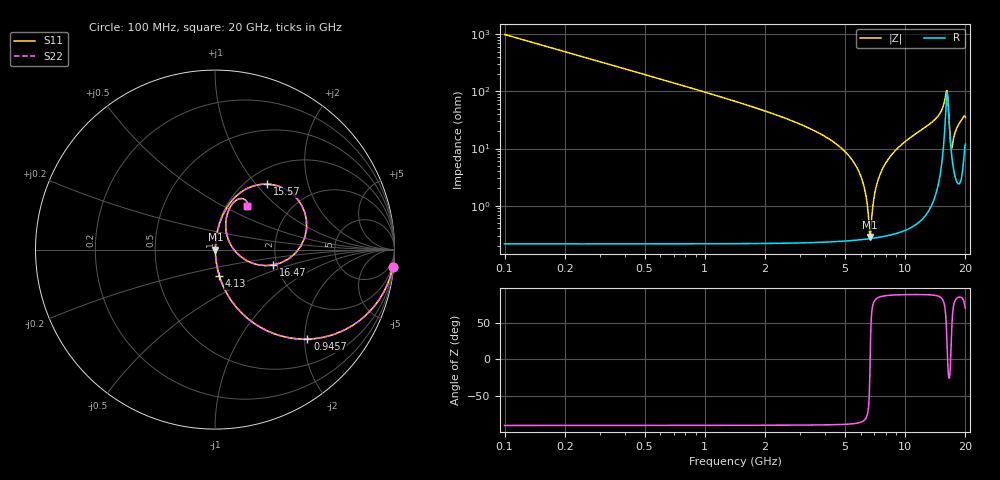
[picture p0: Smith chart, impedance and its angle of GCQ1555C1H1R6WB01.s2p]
!Murata Part Number: GCQ1555C1H1R6WB01
!These Parameters are Measured in Series Mode Connection
!Data Generated on Jan 08, 2026
!  o--ll--o
!Port1  Port2
!  o------o
!Operation Temp=25[degC], DC Bias Voltage=0[V]
!Freq. Start=100[MHz] Stop=20[GHz] 401[Steps]
# Hz S RI R 50
!Freq.(Hz) S11(Real) S11(Imag) S21(Real) S21(Imag) S12(Real) S12(Imag) S22(Real) S22(Imag)
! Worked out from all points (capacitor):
!   401 points, 100 MHz to 20 GHz, reference 50 ohm
!   read as one part in series: C = 1.6 pF near 199.5 MHz
!   lowest |Z| = 284 mohm at 6.667 GHz (marker M1)
!   series resonance near 6.69 GHz, so ESL is about 350 pH
!   S11 on the Smith chart (normalised r, x): 100 MHz: 1, -20; 945.8 MHz: 1.00, -2.06; 4.13 GHz: 1.00, -0.30; 15.57 GHz: 1.23, +1.15; 16.47 GHz: 1.91, -0.37; 20 GHz: 1.24, +0.66
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1e8  0.99 -0.0995  0.01 0.0995  0.01 0.0995  0.99 -0.0995
4.4825e8  0.8297 -0.3754  0.1703 0.3754  0.1703 0.3754  0.8297 -0.3754
9.4575e8  0.5153 -0.4987  0.4847 0.4987  0.4847 0.4987  0.5153 -0.4987
1.891e9  0.1915 -0.3912  0.8085 0.3912  0.8085 0.3912  0.1915 -0.3912
3.43325e9  0.046 -0.2044  0.954 0.2044  0.954 0.2044  0.046 -0.2044
4.12975e9  0.0243 -0.1465  0.9757 0.1465  0.9757 0.1465  0.0243 -0.1465
5.9705e9  0.00371 -0.0344  0.9963 0.0344  0.9963 0.0344  0.00371 -0.0344
6.3685e9  0.00281 -0.0149  0.9972 0.0149  0.9972 0.0149  0.00281 -0.0149
6.667e9  0.00264 -0.00103  0.9974 0.00103  0.9974 0.00103  0.00264 -0.00103
6.7665e9  0.00266 0.00347  0.9973 -0.00347  0.9973 -0.00347  0.00266 0.00347
7.065e9  0.00299 0.0166  0.997 -0.0166  0.997 -0.0166  0.00299 0.0166
7.61225e9  0.00441 0.0396  0.9956 -0.0396  0.9956 -0.0396  0.00441 0.0396
8.5575e9  0.00901 0.0766  0.991 -0.0766  0.991 -0.0766  0.00901 0.0766
1.005e10  0.0211 0.1306  0.9789 -0.1306  0.9789 -0.1306  0.0211 0.1306
1.338325e10  0.0781 0.2521  0.9219 -0.2521  0.9219 -0.2521  0.0781 0.2521
1.557225e10  0.2914 0.3644  0.7086 -0.3644  0.7086 -0.3644  0.2914 0.3644
1.61195e10  0.5095 0.1638  0.4905 -0.1638  0.4905 -0.1638  0.5095 0.1638
1.646775e10  0.3235 -0.0859  0.6765 0.0859  0.6765 0.0859  0.3235 -0.0859
1.67165e10  0.1587 -0.0507  0.8413 0.0507  0.8413 0.0507  0.1587 -0.0507
1.706475e10  0.0759 0.0514  0.9241 -0.0514  0.9241 -0.0514  0.0759 0.0514
1.815925e10  0.0721 0.209  0.9279 -0.209  0.9279 -0.209  0.0721 0.209
2e10  0.178 0.2413  0.822 -0.2413  0.822 -0.2413  0.178 0.2413
